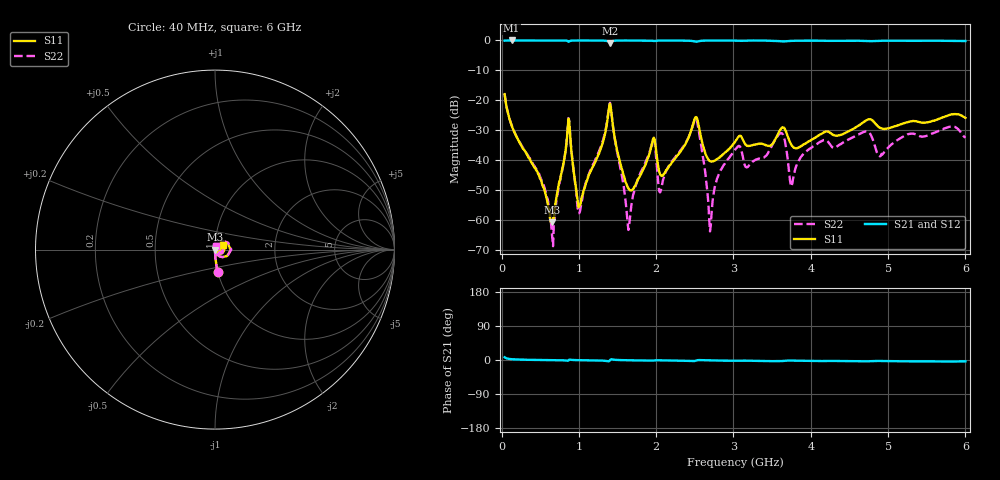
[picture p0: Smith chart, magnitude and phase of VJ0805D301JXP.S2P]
! VJ0805D271JXP
! DATE 03/14/2022  09:39
! CAPACITORS MOUNTED IN SERIES ON 25 MIL THICK MICROSTRIP SUBSTRATE
# GHz  S  MA  R  50.00
!  FREQ  S11M  S11A  S21M  S21A  S12M  S12A  S22M  S22A
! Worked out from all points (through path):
!   600 points, 40 MHz to 6 GHz, reference 50 ohm
!   highest |S21| = 0.00 dB at 129.6 MHz (marker M1); lowest = -0.8 dB at 1.403 GHz (marker M2)
!   lowest |S11| = -60.9 dB at 656.9 MHz (marker M3), VSWR 1.00, Z = 50.1 + j0.00655 ohm
!   |S11| at or under -10 dB: start of sweep to end of sweep
!   |S22| runs from -68.9 to -17.8 dB; largest |S21 - S12| = 0.0049
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0.04  0.1266 -82.5  0.9921 7.2  0.9908 7.3  0.1282 -82.9
0.12955  0.03812 -88.2  1 2.2  0.9987 2.1  0.0389 -87.3
0.5176  0.004361 -83.5  0.9993 0.0  0.9999 0.0  0.004585 -84.4
0.6569  0.0009051 4.1  0.9995 -0.3  0.9999 -0.3  0.0004996 -20.7
0.86585  0.04911 18.9  0.9535 -1.4  0.9548 -1.5  0.05021 21.6
0.98525  0.002073 -37.3  0.9986 -0.4  0.9988 -0.4  0.001557 -38.7
1.035  0.002353 39.3  0.9989 -0.6  0.9992 -0.6  0.001946 55.6
1.40315  0.08775 -2.0  0.911 -0.6  0.9119 -0.7  0.09072 0.5
1.64195  0.00333 -25.1  0.9984 -0.7  0.9988 -0.7  0.0006745 6.1
1.9504  0.01994 37.3  0.9871 -1.7  0.988 -1.8  0.01976 57.6
2.03  0.007338 -21.4  0.9945 -0.9  0.9955 -0.9  0.003797 -1.1
2.5076  0.05167 13.1  0.9546 -2.2  0.956 -2.3  0.04793 24.5
2.7066  0.009446 -8.5  0.9964 -1.3  0.9973 -1.3  0.0007815 60.6
2.8061  0.01072 17.1  0.9969 -1.6  0.9981 -1.7  0.005541 97.1
3.025  0.02045 29.7  0.9934 -2.1  0.9946 -2.2  0.01507 80.2
3.1842  0.01715 7.3  0.9955 -1.8  0.9973 -1.9  0.007612 64.9
3.622  0.03419 19.2  0.9663 -2.8  0.9678 -2.9  0.02817 48.4
3.75135  0.01768 -5.6  0.985 -1.6  0.9863 -1.6  0.003607 57.5
4.02  0.02213 33.1  0.9933 -2.4  0.9946 -2.6  0.0165 97.4
4.7165  0.04605 32.8  0.9798 -3.5  0.9818 -3.5  0.03004 69.7
5.015  0.03411 28.9  0.9913 -2.9  0.9924 -3.0  0.01678 99.3
6.00005  0.05064 27.3  0.9808 -3.5  0.982 -3.6  0.02349 73.2
